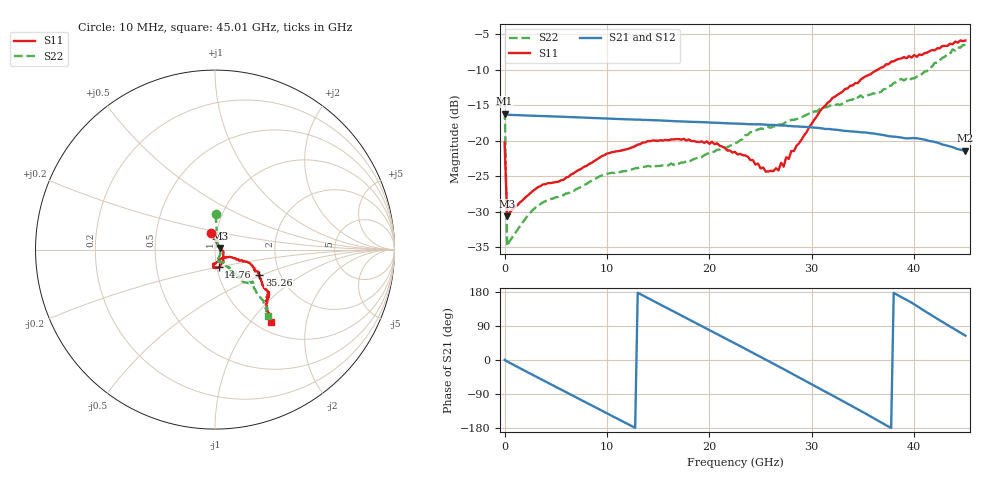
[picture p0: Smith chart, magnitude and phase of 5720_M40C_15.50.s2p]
! Device:  ADRF5720
! Description: 0.5dB LSB GaAs MMIC 6-bit Digital Attenuator
! Frequency:  0.000009 -  40 GHz
! Ports:
!	RF1	= Port 1
!	RF2	= Port 2
! Vdd:  3.3 Volt
! Vss:  -3.3 Volt
! Control:  0/3.3 Volt
! State:  15.50 dB attenuation
! Data:  The device was measured using G-S-G Probes on a matrix board.
!  Data was collected using an calibrated 4 port network analyzer.
!  The reference plane for this measurement is at the launchers.
! Note:  Analog Devices supplies this data as a sample of measured data
!  for this product.  Your particular data for this product may vary.
!  Data was taken at -40 degrees C.
!  Analog Devices reserves the right to change this data at anytime.
# GHZ S DB R 45.0
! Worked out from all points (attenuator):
!   181 points, 10 MHz to 45.01 GHz, reference 45 ohm
!   highest |S21| = -16.16 dB at 10 MHz (marker M1); lowest = -21.4 dB at 45.01 GHz (marker M2)
!   lowest |S11| = -30.6 dB at 260 MHz (marker M3), VSWR 1.06, Z = 47.6 + j0.834 ohm
!   |S11| at or under -10 dB: start of sweep to 36.43 GHz
!   |S22| runs from -34.8 to -6.5 dB; largest |S21 - S12| = 0.00058
!   S11 on the Smith chart (normalised r, x): 10 MHz: 0.93, +0.18; 14.76 GHz: 1.02, -0.20; 35.26 GHz: 1.57, -0.47; 45.01 GHz: 1.17, -1.27
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0.01  -20.23 104.8  -16.16 0.3  -16.18 0.3  -14.08 89.2
0.26  -30.60 17.3  -16.34 -3.9  -16.36 -3.9  -34.83 26.0
3.26  -26.52 -13.8  -16.50 -46.4  -16.53 -46.4  -29.07 -30.6
5.76  -25.50 -30.4  -16.62 -81.4  -16.65 -81.4  -27.66 -50.2
7.76  -23.66 -44.4  -16.74 -109.3  -16.76 -109.3  -26.24 -64.6
11.51  -21.34 -62.3  -16.95 -161.7  -16.97 -161.7  -24.30 -74.6
14.76  -20.00 -78.3  -17.12 152.8  -17.14 152.7  -23.57 -75.2
15.26  -19.92 -80.4  -17.14 145.7  -17.16 145.6  -23.52 -74.9
20.26  -20.13 -95.3  -17.44 75.4  -17.46 75.3  -21.62 -59.1
22.76  -21.92 -96.9  -17.59 40.2  -17.61 40.1  -20.20 -56.8
25.51  -24.33 -64.3  -17.74 1.0  -17.76 0.8  -18.20 -52.9
26.76  -24.16 -44.9  -17.84 -17.0  -17.86 -17.1  -17.69 -51.8
27.01  -23.09 -42.2  -17.85 -20.4  -17.87 -20.6  -17.70 -53.2
27.26  -23.63 -39.8  -17.86 -24.1  -17.88 -24.2  -17.57 -51.6
27.51  -22.33 -35.8  -17.86 -27.8  -17.88 -27.9  -17.35 -52.8
27.76  -22.55 -33.2  -17.92 -31.5  -17.94 -31.6  -17.18 -51.2
30.26  -17.02 -22.4  -18.15 -67.8  -18.17 -68.0  -15.84 -52.5
32.01  -14.00 -21.5  -18.40 -93.5  -18.42 -93.6  -15.06 -50.0
35.26  -10.94 -29.3  -18.82 -141.3  -18.85 -141.5  -13.70 -48.0
37.76  -8.85 -38.4  -19.39 -179.3  -19.41 -179.5  -12.24 -48.0
40.26  -8.18 -42.6  -19.64 142.7  -19.66 142.5  -10.97 -40.9
45.01  -5.88 -52.1  -21.40 64.3  -21.44 64.1  -6.51 -51.4
